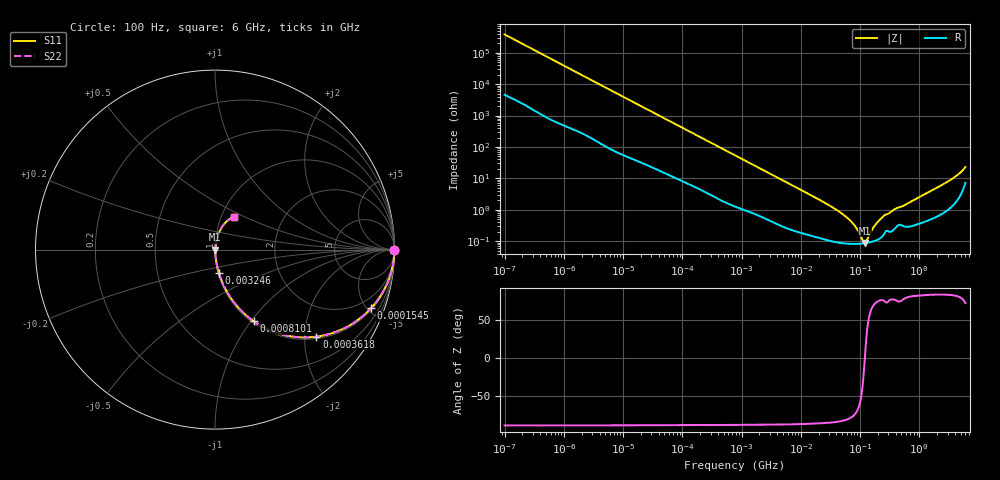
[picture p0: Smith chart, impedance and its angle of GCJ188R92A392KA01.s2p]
!Murata Part Number: GCJ188R92A392KA01
!These Parameters are Measured in Series Mode Connection
!Data Generated on Mar 13, 2026
!  o--ll--o
!Port1  Port2
!  o------o
!Operation Temp=25[degC], DC Bias Voltage=0[V]
!Freq. Start=100[Hz] Stop=6[GHz] 401[Steps]
# Hz S RI R 50
!Freq.(Hz) S11(Real) S11(Imag) S21(Real) S21(Imag) S12(Real) S12(Imag) S22(Real) S22(Imag)
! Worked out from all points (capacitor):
!   401 points, 100 Hz to 6 GHz, reference 50 ohm
!   read as one part in series: C = 4.16 nF near 109 Hz
!   lowest |Z| = 87.3 mohm at 122 MHz (marker M1)
!   series resonance near 120.5 MHz, so ESL is about 420 pH
!   S11 on the Smith chart (normalised r, x): 100 Hz: open; 154.5 kHz: 1.11, -5.28; 361.8 kHz: 1.05, -2.28; 810.1 kHz: 1.02, -1.03; 3.246 MHz: 1.01, -0.26; 6 GHz: 1.14, +0.44
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100  1 -0.000262  3.2e-06 0.000262  3.2e-06 0.000262  1 -0.000262
2008  0.9999 -0.00514  9.91e-05 0.00514  9.91e-05 0.00514  0.9999 -0.00514
12592  0.9985 -0.0317  0.00147 0.0317  0.00147 0.0317  0.9985 -0.0317
40335  0.9883 -0.0991  0.0117 0.0991  0.0117 0.0991  0.9883 -0.0991
86348  0.9529 -0.2022  0.0471 0.2022  0.0471 0.2022  0.9529 -0.2022
154540  0.8695 -0.3265  0.1305 0.3265  0.1305 0.3265  0.8695 -0.3265
361830  0.5646 -0.4851  0.4354 0.4851  0.4354 0.4851  0.5646 -0.4851
774597  0.2298 -0.4091  0.7702 0.4091  0.7702 0.4091  0.2298 -0.4091
810067  0.215 -0.3991  0.785 0.3991  0.785 0.3991  0.215 -0.3991
1449809  0.0839 -0.2636  0.9161 0.2636  0.9161 0.2636  0.0839 -0.2636
3245845  0.021 -0.1283  0.979 0.1283  0.979 0.1283  0.021 -0.1283
1.555665e7  0.00222 -0.0276  0.9978 0.0276  0.9978 0.0276  0.00222 -0.0276
3.64232e7  0.00108 -0.0111  0.9989 0.0111  0.9989 0.0111  0.00108 -0.0111
5.960426e7  0.000868 -0.00568  0.9991 0.00568  0.9991 0.00568  0.000868 -0.00568
8.154455e7  0.000828 -0.00298  0.9992 0.00298  0.9992 0.00298  0.000828 -0.00298
1.115611e8  0.000849 -0.000574  0.9992 0.000574  0.9992 0.000574  0.000849 -0.000574
1.220122e8  0.000867 9.56e-05  0.9991 -9.56e-05  0.9991 -9.56e-05  0.000867 9.56e-05
1.909225e8  0.00109 0.00359  0.9989 -0.00359  0.9989 -0.00359  0.00109 0.00359
2.497637e8  0.00163 0.00609  0.9984 -0.00609  0.9984 -0.00609  0.00163 0.00609
3.124326e8  0.00204 0.00759  0.998 -0.00759  0.998 -0.00759  0.00204 0.00759
2.802721e9  0.0138 0.0706  0.9862 -0.0706  0.9862 -0.0706  0.0138 0.0706
6e9  0.1046 0.183  0.8954 -0.183  0.8954 -0.183  0.1046 0.183
